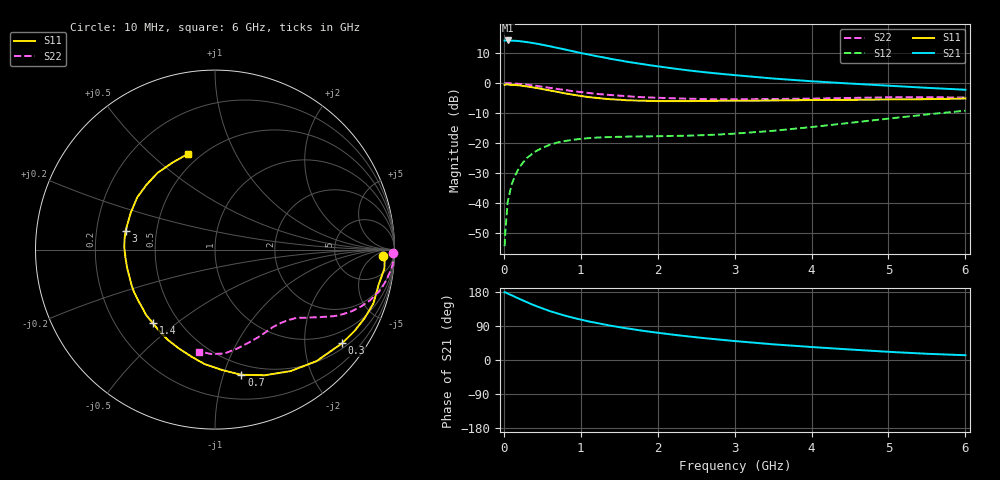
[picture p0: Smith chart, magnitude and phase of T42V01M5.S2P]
! Infineon Technologies  Discrete & RF Semiconductors
! BFR182T
! Si NPN RF Bipolar Junction Transistor in SC75
! VCE = 2 V  IC = 1.5 mA
! Common Emitter S-Parameters:  October  1999
# GHz  S  MA  R  50
!  f  S11  S21  S12  S22
! GHz  MAG  ANG  MAG  ANG  MAG  ANG  MAG  ANG
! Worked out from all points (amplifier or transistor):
!   36 points, 10 MHz to 6 GHz, reference 50 ohm
!   highest |S21| = 14.2 dB at 50 MHz (marker M1)
!   |S21| within 3 dB of that: start of sweep to 792.5 MHz
!   unconditionally stable (mu >= 1): 2.14 GHz to 4.462 GHz
!   at 250 MHz: K = 0.12, MSG = 20.2 dB, |S12| = -26.5 dB
!   at 1.4 GHz: K = 0.70, MSG = 13.0 dB, |S12| = -18.0 dB
!   at 6 GHz: K = 0.84, MSG = 3.5 dB, |S12| = -9.2 dB
!   S11 on the Smith chart (normalised r, x): 10 MHz: 22, -13; 300 MHz: 0.63, -2.93; 700 MHz: 0.41, -1.15; 1.4 GHz: 0.36, -0.41; 3 GHz: 0.33, +0.09; 6 GHz: 0.43, +0.66
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0.01  0.9361 -2.3  5.125 178.6  0.0019 78.6  0.9911 -1.2
0.02  0.9463 -1.2  5.129 178.5  0.0034 97.2  0.9999 -1.1
0.05  0.9498 -6.4  5.154 175.4  0.0104 87.1  0.9951 -2.6
0.1  0.9325 -12.0  5.11 171.0  0.0201 84.3  0.9927 -5.1
0.15  0.9321 -18.8  5.083 166.1  0.0293 78.9  0.9818 -7.5
0.2  0.9167 -24.7  5.029 161.5  0.0389 76.6  0.9716 -9.8
0.3  0.88 -36.3  4.837 152.5  0.0563 70.0  0.9436 -14.3
0.4  0.8402 -47.7  4.622 143.9  0.071 63.5  0.9083 -18.2
0.5  0.7973 -58.1  4.371 136.3  0.0832 58.5  0.8706 -21.5
0.6  0.753 -68.4  4.117 129.0  0.0938 53.8  0.834 -24.4
0.7  0.7128 -78.1  3.862 122.7  0.1024 50.4  0.7977 -26.8
0.9  0.6406 -95.2  3.397 111.5  0.1132 44.0  0.7336 -30.6
1.1  0.5853 -110.4  3.004 101.8  0.1206 39.9  0.6855 -33.4
1.4  0.5364 -130.1  2.523 90.2  0.1258 36.1  0.6317 -37.0
1.8  0.5092 -152.4  2.082 77.3  0.1291 35.3  0.5833 -41.2
2.2  0.5001 -168.2  1.76 66.8  0.1315 37.3  0.5595 -45.4
2.6  0.5052 178.8  1.526 57.8  0.1355 41.1  0.5433 -50.6
3  0.509 168.1  1.36 50.0  0.1436 45.7  0.539 -55.4
3.5  0.5124 156.3  1.194 41.4  0.1599 51.4  0.5435 -62.6
4.5  0.5256 136.7  0.984 27.7  0.2172 57.9  0.5653 -77.4
5.5  0.5397 115.8  0.835 16.4  0.2999 57.1  0.5822 -91.9
6  0.5537 106.0  0.775 12.6  0.3468 54.3  0.5746 -98.7
